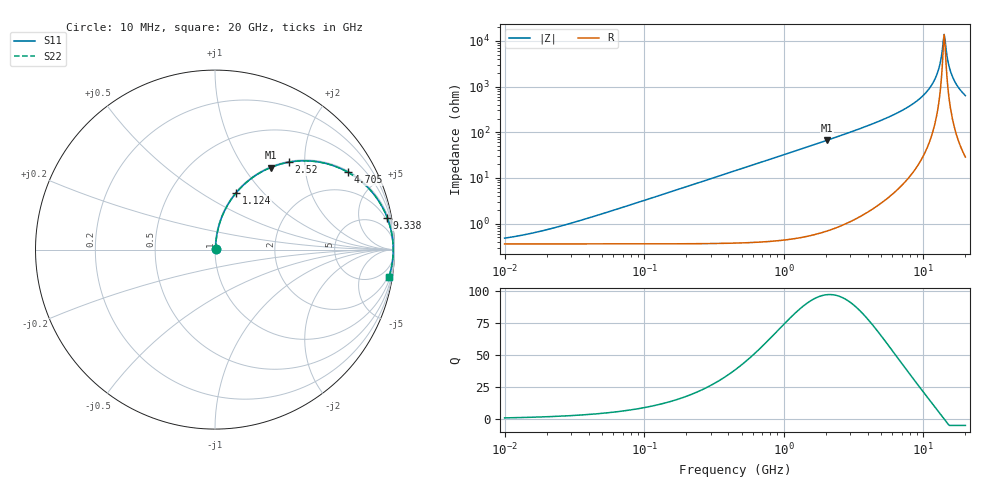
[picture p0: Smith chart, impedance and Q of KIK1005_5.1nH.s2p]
!version-3
!date-01.2023
!Series
# Hz S RI R 50
!Freq ReS11 ImS11 ReS21 ImS21 ReS12 ImS12 ReS22 ImS22
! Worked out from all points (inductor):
!   500 points, 10 MHz to 20 GHz, reference 50 ohm
!   read as one part in series: L = 5.1 nH near 33.82 MHz
!   highest Q = 96.9 at 2.036 GHz (marker M1), where L = 5.21 nH
!   self-resonance near 14.09 GHz
!   S11 on the Smith chart (normalised r, x): 10 MHz: 1.01, +0.01; 1.124 GHz: 1.01, +0.72; 2.52 GHz: 1.02, +1.67; 4.705 GHz: 1.05, +3.39; 9.338 GHz: 1, +11; 20 GHz: 2, -13
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1e7  0.0036 0.00318  0.9964 -0.00318  0.9964 -0.00318  0.0036 0.00318
3.59488e7  0.00372 0.0114  0.9963 -0.0114  0.9963 -0.0114  0.00372 0.0114
1.272781e8  0.00524 0.0404  0.9948 -0.0404  0.9948 -0.0404  0.00524 0.0404
4.506326e8  0.024 0.1405  0.976 -0.1405  0.976 -0.1405  0.024 0.1405
1.123932e9  0.1192 0.3178  0.8808 -0.3178  0.8808 -0.3178  0.1192 0.3178
1.595481e9  0.214 0.4048  0.786 -0.4048  0.786 -0.4048  0.214 0.4048
2.035806e9  0.3092 0.457  0.6908 -0.457  0.6908 -0.457  0.3092 0.457
2.51971e9  0.4111 0.4868  0.5889 -0.4868  0.5889 -0.4868  0.4111 0.4868
4.705192e9  0.739 0.4319  0.261 -0.4319  0.261 -0.4319  0.739 0.4319
5.648861e9  0.8186 0.3767  0.1814 -0.3767  0.1814 -0.3767  0.8186 0.3767
9.338249e9  0.9593 0.1788  0.0407 -0.1788  0.0407 -0.1788  0.9593 0.1788
1.087473e10  0.9796 0.1133  0.0204 -0.1133  0.0204 -0.1133  0.9796 0.1133
1.209833e10  0.9882 0.067  0.0118 -0.067  0.0118 -0.067  0.9882 0.067
1.285839e10  0.9912 0.0405  0.00884 -0.0405  0.00884 -0.0405  0.9912 0.0405
1.387596e10  0.9928 0.00726  0.00722 -0.00726  0.00722 -0.00726  0.9928 0.00726
1.408894e10  0.9928 0.000617  0.00716 -0.000617  0.00716 -0.000617  0.9928 0.000617
1.452476e10  0.9927 -0.0127  0.00731 0.0127  0.00731 0.0127  0.9927 -0.0127
1.497406e10  0.9922 -0.026  0.00782 0.026  0.00782 0.026  0.9922 -0.026
1.543725e10  0.9913 -0.0392  0.00868 0.0392  0.00868 0.0392  0.9913 -0.0392
1.615905e10  0.9893 -0.0591  0.0107 0.0591  0.0107 0.0591  0.9893 -0.0591
1.770548e10  0.983 -0.0989  0.017 0.0989  0.017 0.0989  0.983 -0.0989
2e10  0.9692 -0.1516  0.0308 0.1516  0.0308 0.1516  0.9692 -0.1516
